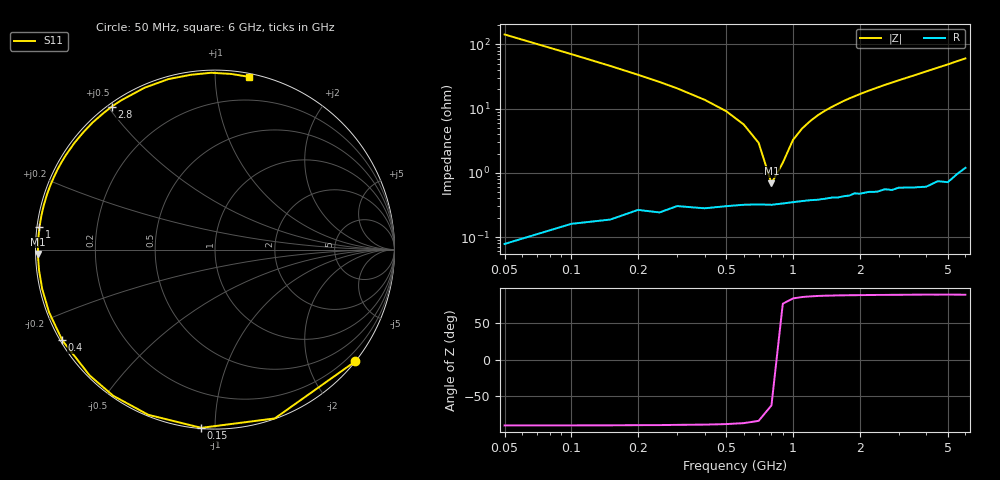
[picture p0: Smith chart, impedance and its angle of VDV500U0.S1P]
! Infineon Technologies  Discrete & RF Semiconductors
! BBY 55-03
! Si Tuning Diode in SOD323
! VR = 0.5 V
! S-Parameters:  June  1999
# GHz  S  MA  R  50
!  f  S11
! GHz  MAG  ANG
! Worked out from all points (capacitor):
!   34 points, 50 MHz to 6 GHz, reference 50 ohm
!   read as one part to ground: C = 22.2 pF near 50 MHz
!   lowest |Z| = 689 mohm at 800 MHz (marker M1)
!   series resonance near 830.4 MHz, so ESL is about 1.7 nH
!   S11 on the Smith chart (normalised r, x): 50 MHz: 0.00, -2.86; 150 MHz: 0.00, -0.93; 400 MHz: 0.01, -0.27; 1 GHz: 0.01, +0.06; 2.8 GHz: 0.01, +0.51; 6 GHz: 0.02, +1.21
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0.05  0.9997 -38.5
0.1  0.9979 -70.5
0.15  0.996 -94.4
0.2  0.9927 -112.0
0.25  0.9924 -124.9
0.3  0.9897 -134.9
0.4  0.9896 -149.3
0.5  0.9883 -159.3
0.6  0.9875 -167.1
0.7  0.9872 -173.3
0.8  0.9873 -178.6
0.9  0.9868 176.8
1  0.9862 172.6
1.1  0.9857 168.8
1.3  0.9852 161.9
1.4  0.9848 158.8
1.6  0.9845 153.1
1.8  0.9838 147.7
2  0.9831 142.8
2.4  0.9829 133.9
2.8  0.983 125.9
3  0.9821 122.1
3.5  0.9836 113.5
4  0.9847 105.3
4.5  0.9833 97.9
5  0.9855 91.2
5.5  0.9828 84.7
6  0.9808 79.0
